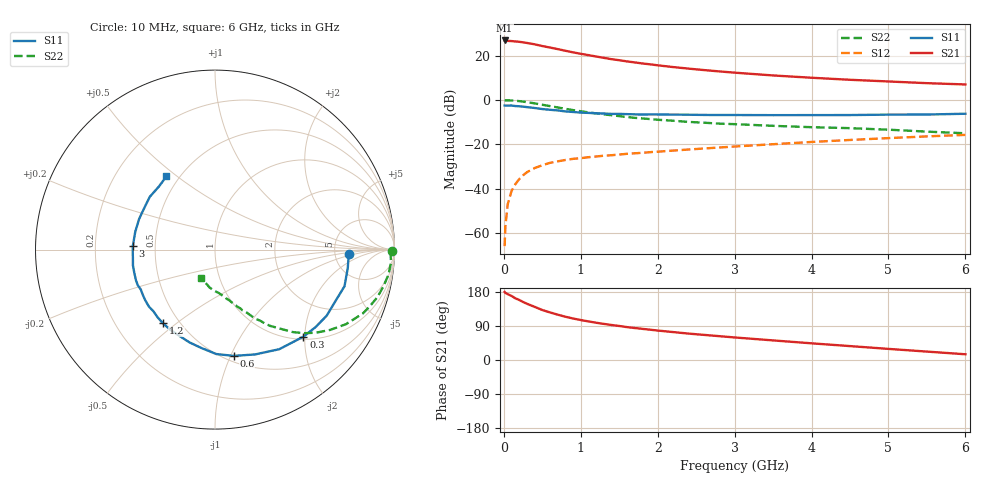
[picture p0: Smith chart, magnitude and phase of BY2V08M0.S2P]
! SIEMENS Small Signal Semiconductors
! BFY420
! Si NPN RF SIEGET Grounded Emitter Transistor in MICRO-X
! VCE = 2 V  IC = 8 mA
! Common Emitter S-Parameters:  October  1996
# GHz  S  MA  R  50
!  f  S11  S21  S12  S22
! GHz  MAG  ANG  MAG  ANG  MAG  ANG  MAG  ANG
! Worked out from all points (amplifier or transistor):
!   36 points, 10 MHz to 6 GHz, reference 50 ohm
!   highest |S21| = 26.9 dB at 10 MHz (marker M1)
!   |S21| within 3 dB of that: start of sweep to 570.3 MHz
!   unconditionally stable (mu >= 1): 2.686 GHz to end of sweep
!   at 250 MHz: K = 0.16, MSG = 30.0 dB, |S12| = -34.0 dB
!   at 1.4 GHz: K = 0.68, MSG = 21.7 dB, |S12| = -24.9 dB
!   at 6 GHz: K = 1.11, MAG = 9.3 dB, |S12| = -15.8 dB
!   S11 on the Smith chart (normalised r, x): 10 MHz: 6.91, -0.74; 300 MHz: 1.06, -1.97; 600 MHz: 0.55, -1.03; 1.2 GHz: 0.41, -0.45; 3 GHz: 0.37, +0.02; 6 GHz: 0.43, +0.46
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0.01  0.7497 -1.8  22.13 179.5  0.0005 89.5  0.9837 -0.6
0.02  0.7453 -3.2  21.97 177.1  0.0014 89.3  0.9786 -1.5
0.05  0.7468 -7.8  21.61 173.7  0.0044 89.6  0.9834 -4.1
0.1  0.7499 -15.8  21.46 169.1  0.0088 83.2  0.9765 -8.3
0.15  0.7301 -23.0  21 162.8  0.0126 77.6  0.9603 -12.3
0.2  0.723 -30.6  20.64 158.4  0.0163 75.5  0.9436 -16.2
0.25  0.7078 -37.5  20.07 153.1  0.0199 71.2  0.9193 -20.0
0.3  0.6911 -44.6  19.45 148.4  0.0234 69.4  0.897 -23.4
0.4  0.6603 -57.2  18.11 140.3  0.029 64.2  0.8394 -29.7
0.5  0.6252 -69.1  16.55 131.9  0.0336 59.3  0.7821 -34.9
0.6  0.6014 -80.0  15.31 125.6  0.0381 55.4  0.728 -39.5
0.8  0.5528 -98.1  12.95 114.2  0.0442 50.8  0.6325 -46.6
0.9  0.5362 -105.4  11.91 109.5  0.0469 48.7  0.5916 -49.1
1.1  0.5114 -119.3  10.32 101.8  0.0511 46.8  0.526 -54.0
1.2  0.5022 -125.3  9.601 98.3  0.053 46.2  0.4984 -55.9
1.6  0.4801 -144.3  7.446 86.8  0.0609 44.1  0.4139 -61.8
2.2  0.4678 -164.1  5.544 73.7  0.0721 43.0  0.3402 -68.7
3  0.4582 177.5  4.147 59.5  0.0891 41.3  0.285 -76.0
3.5  0.4553 167.3  3.587 51.7  0.1004 39.4  0.261 -80.5
4.5  0.4574 149.2  2.862 36.7  0.1252 33.8  0.2314 -90.1
5.5  0.4703 131.6  2.402 22.2  0.1508 26.6  0.1932 -105.4
6  0.4896 123.6  2.246 15.1  0.1631 22.5  0.1773 -115.5
